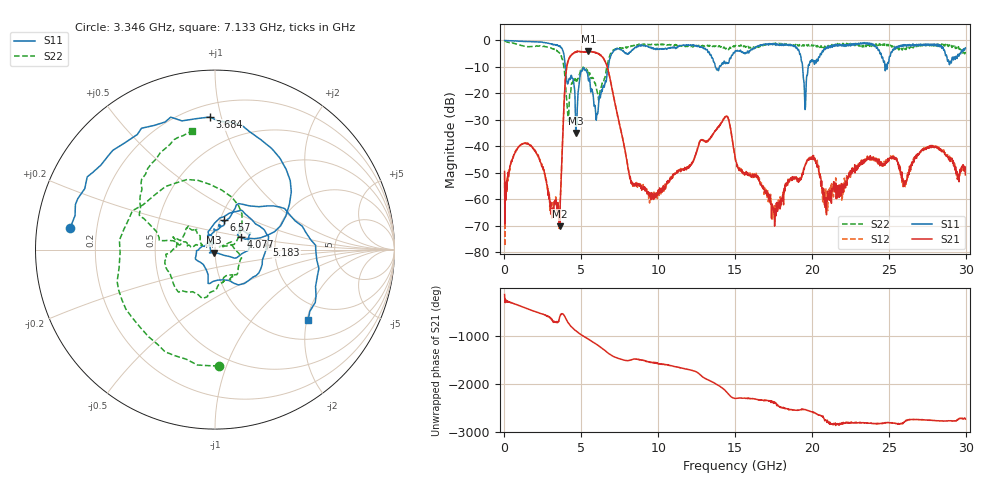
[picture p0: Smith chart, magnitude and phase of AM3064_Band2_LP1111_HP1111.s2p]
# Hz S DB R 50.0
!freq dBS11 angS11 dBS21 angS21 dBS12 angS12 dBS22 angS22
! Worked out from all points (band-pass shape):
!   1600 points, 10 MHz to 29.98 GHz, reference 50 ohm
!   highest |S21| = -4.11 dB at 5.464 GHz (marker M1); lowest = -70.3 dB at 3.609 GHz (marker M2)
!   |S21| within 3 dB of the highest: 4.18 GHz to 6.471 GHz (2.292 GHz wide, 43 % of centre)
!   lowest |S11| = -35.0 dB at 4.64 GHz (marker M3), VSWR 1.04, Z = 49.3 - j1.64 ohm
!   |S11| at or under -10 dB: 3.959 GHz to 6.762 GHz (2.803 GHz wide, 52.3 % of centre); 13.72 GHz to 13.98 GHz (260.3 MHz wide, 1.88 % of centre); 19.39 GHz to 19.75 GHz (362.2 MHz wide, 1.85 % of centre)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
!   |S22| runs from -30.5 to -0.1 dB; largest |S21 - S12| = 0.014
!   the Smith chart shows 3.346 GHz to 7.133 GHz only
!   S11 on the Smith chart (normalised r, x): 3.346 GHz: 0.10, +0.07; 3.684 GHz: 0.28, +0.92; 4.077 GHz: 1.32, +0.19; 5.183 GHz: 1.81, +0.11; 6.57 GHz: 1.04, +0.35; 7.133 GHz: 1.48, -2.04
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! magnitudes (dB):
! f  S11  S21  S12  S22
! 10 MHz  0.0  -49.5  -50.6  -0.1
! 1.453 GHz  -0.4  -38.9  -38.9  -2.3
! 3.346 GHz  -1.8  -60.2  -60.2  -3.8
! 3.609 GHz  -2.3  -70.3  -64.9  -5.3
! 3.684 GHz  -2.6  -53.1  -53.1  -5.9
! 4.077 GHz  -16.0  -9.2  -9.2  -24.8
! 4.64 GHz  -35.0  -4.5  -4.4  -15.4
! 5.015 GHz  -11.7  -4.3  -4.2  -11.4
! 5.183 GHz  -10.7  -4.3  -4.3  -10.5
! 5.464 GHz  -15.2  -4.1  -4.0  -13.3
! 5.971 GHz  -30.1  -4.7  -4.6  -17.7
! 6.57 GHz  -15.4  -8.3  -8.2  -13.4
! 7.133 GHz  -3.7  -22.3  -22.1  -3.5
! 8.257 GHz  -3.9  -53.1  -53.7  -2.0
! 10 GHz  -3.4  -58.4  -57.3  -1.7
! 14.37 GHz  -8.8  -28.8  -28.8  -3.2
! 15 GHz  -4.1  -44.5  -44.2  -2.1
! 17.52 GHz  -1.4  -64.8  -62.5  -1.2
! 19.99 GHz  -7.3  -44.9  -44.3  -1.7
! 20.91 GHz  -2.7  -63.4  -55.9  -2.6
! 25 GHz  -8.2  -44.8  -44.8  -1.6
! 29.98 GHz  -2.8  -50.8  -49.2  -4.3
